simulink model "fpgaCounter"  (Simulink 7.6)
settings: Solver=FixedStepDiscrete  StartTime=0.0  StopTime=0.01  RelTol=1e-3
undefined symbols (not defined in the file or in its folder): Bitfile_Generator, usrp_FPGA
libraries: dspsrcs4 x2, simulink x2

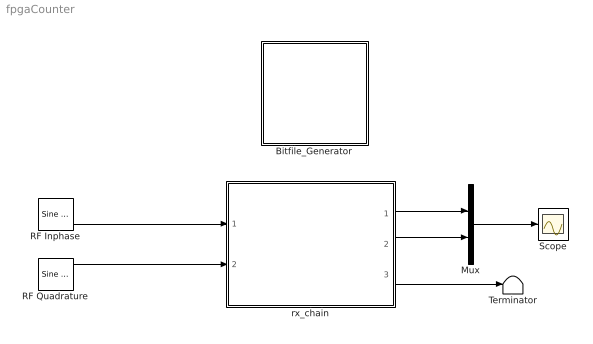
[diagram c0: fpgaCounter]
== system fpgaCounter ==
  Bitfile_Generator : Subsystem  AncestorBlock=usrp_FPGA/Bitfile_Generator
  Mux : Mux  Inputs=2
  RF Inphase : dspsrcs4/Sine Wave  Amplitude=1  Frequency=8e6  Phase=0  SampleMode=Discrete  OutComplex=Real  CompMethod=Table lookup  TableSize=Speed  SampleTime=1/64e6  SamplesPerFrame=1  ResetState=Restart at time zero  dataType=Fixed-point  wordLen=16  udDataType=fixdt('ufix16')  fracBitsMode=Best precision  numFracBits=14  OutDataTypeStr=fixdt(1,16)  LastOutDataTypeStr=fixdt(1,16)
  RF Quadrature : dspsrcs4/Sine Wave  Amplitude=1  Frequency=8e6  Phase=0  SampleMode=Discrete  OutComplex=Real  CompMethod=Table lookup  TableSize=Speed  SampleTime=1/64e6  SamplesPerFrame=1  ResetState=Restart at time zero  dataType=Fixed-point  wordLen=16  udDataType=fixdt('ufix16')  fracBitsMode=Best precision  numFracBits=14  OutDataTypeStr=fixdt(1,16)  LastOutDataTypeStr=fixdt(1,16)
  Scope : Scope
  Terminator : Terminator
  rx_chain : Subsystem
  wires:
  RF Inphase/1 -> rx_chain/1(i_in)
  RF Quadrature/1 -> rx_chain/2(q_in)
  rx_chain/1(i_out) -> Mux/1
  rx_chain/2(q_out) -> Mux/2
  rx_chain/3(debug) -> Terminator/1
  Mux/1 -> Scope/1

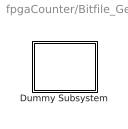
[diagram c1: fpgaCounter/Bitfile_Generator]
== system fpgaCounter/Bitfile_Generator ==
  Dummy Subsystem : Subsystem

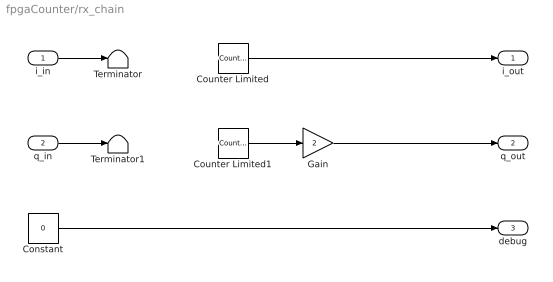
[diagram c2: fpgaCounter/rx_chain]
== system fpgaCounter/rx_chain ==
  i_in : Inport
  q_in : Inport  Port=2
  Constant : Constant  Value=0  OutDataTypeStr=boolean  SampleTime=1/64e6
  Counter Limited : simulink/Sources/Counter Limited  SystemSampleTime=-1  uplimit=2^16-1  tsamp=512/64e6
  Counter Limited1 : simulink/Sources/Counter Limited  SystemSampleTime=-1  uplimit=2^16-1  tsamp=512/64e6
  Gain : Gain  Gain=2  OutDataTypeStr=uint16
  Terminator : Terminator
  Terminator1 : Terminator
  i_out : Outport
  q_out : Outport  Port=2
  debug : Outport  Port=3
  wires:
  Constant/1 -> debug/1
  Counter Limited1/1 -> Gain/1
  Counter Limited/1 -> i_out/1
  Gain/1 -> q_out/1
  i_in/1 -> Terminator/1
  q_in/1 -> Terminator1/1

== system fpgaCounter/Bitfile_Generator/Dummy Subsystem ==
